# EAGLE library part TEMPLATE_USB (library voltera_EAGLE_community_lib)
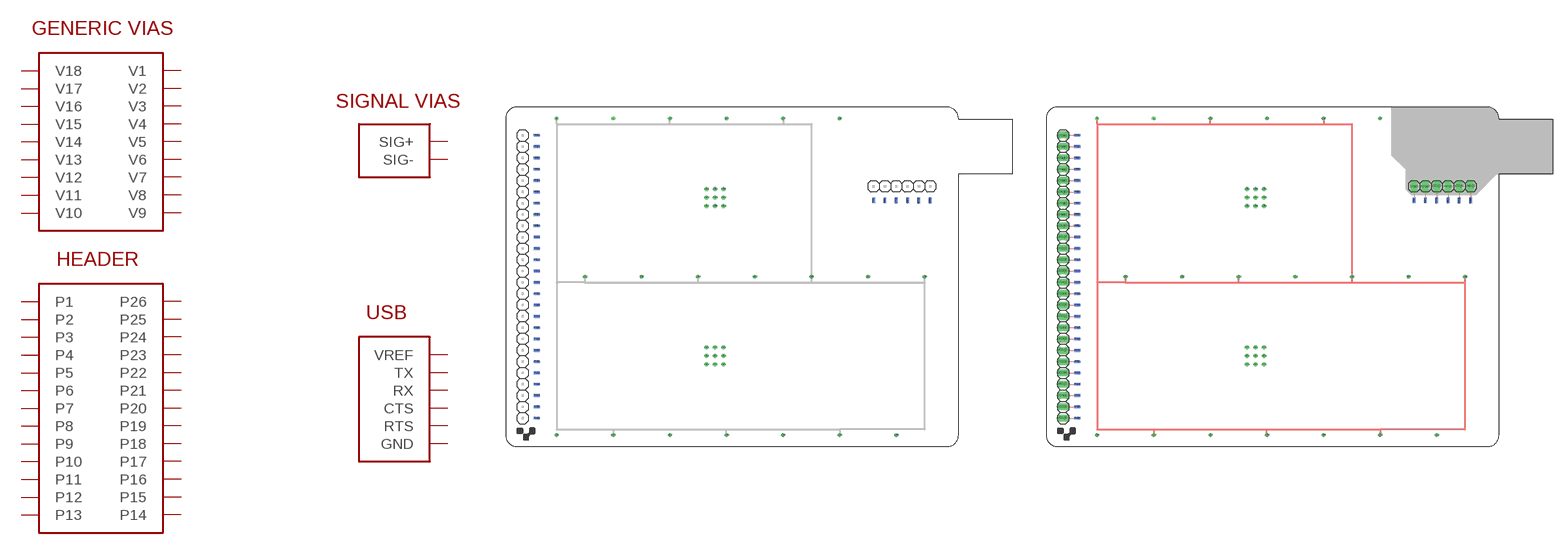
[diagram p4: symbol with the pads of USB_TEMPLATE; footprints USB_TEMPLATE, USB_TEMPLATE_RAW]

Designator prefix -

## TEMPLATE_USB_TEMPLATE  [USB_TEMPLATE]
+  SIG+
+@1  SIG+
+@2  SIG+
+@3  SIG+
+@4  SIG+
+@5  SIG+
+@6  SIG+
+@7  SIG+
+@8  SIG+
+@9  SIG+
-  SIG-
-@1  SIG-
-@2  SIG-
-@3  SIG-
-@4  SIG-
-@5  SIG-
-@6  SIG-
-@7  SIG-
-@8  SIG-
-@9  SIG-
CTS  CTS
CTS1  CTS
GND  GND
GND1  GND
P1  P1
P1@1  P1
P2  P2
P2@1  P2
P3  P3
P3@1  P3
P4  P4
P4@1  P4
P5  P5
P5@1  P5
P6  P6
P6@1  P6
P7  P7
P7@1  P7
P8  P8
P8@1  P8
P9  P9
P9@1  P9
P10  P10
P10@1  P10
P11  P11
P11@1  P11
P12  P12
P12@1  P12
P13  P13
P13@1  P13
P14  P14
P14@1  P14
P15  P15
P15@1  P15
P16  P16
P16@1  P16
P17  P17
P17@1  P17
P18  P18
P18@1  P18
P19  P19
P19@1  P19
P20  P20
P20@1  P20
P21  P21
P21@1  P21
P22  P22
P22@1  P22
P23  P23
P23@1  P23
P24  P24
P24@1  P24
P25  P25
P25@1  P25
P26  P26
P26@1  P26
RTS  RTS
RTS1  RTS
RX  RX
RX1  RX
TX  TX
TX1  TX
VIA1  V1
VIA2  V2
VIA3  V3
VIA4  V4
VIA5  V5
VIA6  V6
VIA7  V7
VIA8  V8
VIA9  V9
VIA10  V10
VIA11  V11
VIA12  V12
VIA13  V13
VIA14  V14
VIA15  V15
VIA16  V16
VIA17  V17
VIA18  V18
VREF  VREF
VREF1  VREF

## TEMPLATE_USBRAW  [USB_TEMPLATE_RAW]
+  SIG+
+@1  SIG+
+@2  SIG+
+@3  SIG+
+@4  SIG+
+@5  SIG+
+@6  SIG+
+@7  SIG+
+@8  SIG+
+@9  SIG+
-  SIG-
-@1  SIG-
-@2  SIG-
-@3  SIG-
-@4  SIG-
-@5  SIG-
-@6  SIG-
-@7  SIG-
-@8  SIG-
-@9  SIG-
CTS  CTS
CTS1  CTS
CTS@2  CTS
GND  GND
GND1  GND
GND@2  GND
P1  P1
P1@1  P1
P1@2  P1
P2  P2
P2@1  P2
P2@2  P2
P3  P3
P3@1  P3
P3@2  P3
P4  P4
P4@1  P4
P4@2  P4
P5  P5
P5@1  P5
P5@2  P5
P6  P6
P6@1  P6
P6@2  P6
P7  P7
P7@1  P7
P7@2  P7
P8  P8
P8@1  P8
P8@2  P8
P9  P9
P9@1  P9
P9@2  P9
P10  P10
P10@1  P10
P10@2  P10
P11  P11
P11@1  P11
P11@2  P11
P12  P12
P12@1  P12
P12@2  P12
P13  P13
P13@1  P13
P13@2  P13
P14  P14
P14@1  P14
P14@2  P14
P15  P15
P15@1  P15
P15@2  P15
P16  P16
P16@1  P16
P16@2  P16
P17  P17
P17@1  P17
P17@2  P17
P18  P18
P18@1  P18
P18@2  P18
P19  P19
P19@1  P19
P19@2  P19
P20  P20
P20@1  P20
P20@2  P20
P21  P21
P21@1  P21
P21@2  P21
P22  P22
P22@1  P22
P22@2  P22
P23  P23
P23@1  P23
P23@2  P23
P24  P24
P24@1  P24
P24@2  P24
P25  P25
P25@1  P25
P25@2  P25
P26  P26
P26@1  P26
P26@2  P26
RTS  RTS
RTS1  RTS
RTS@2  RTS
RX  RX
RX1  RX
RX@2  RX
TX  TX
TX1  TX
TX@2  TX
VIA1  V1
VIA2  V2
VIA3  V3
VIA4  V4
VIA5  V5
VIA6  V6
VIA7  V7
VIA8  V8
VIA9  V9
VIA10  V10
VIA11  V11
VIA12  V12
VIA13  V13
VIA14  V14
VIA15  V15
VIA16  V16
VIA17  V17
VIA18  V18
VREF  VREF
VREF1  VREF
VREF@2  VREF

## Footprint USB_TEMPLATE (pad centres in mm)
drill 0.3 pad 0.8: + 11.43,73.66; +@1 36.83,73.66; +@2 62.23,73.66; +@3 17.78,38.1; +@4 43.18,38.1; +@5 68.58,38.1; +@6 93.98,38.1; +@7 24.13,2.54; +@8 49.53,2.54; +@9 74.93,2.54; - 24.13,73.66; -@1 49.53,73.66; -@2 74.93,73.66; -@3 81.28,38.1; -@4 55.88,38.1; -@5 30.48,38.1; -@6 11.43,2.54; -@7 36.83,2.54; -@8 62.23,2.54; -@9 87.63,2.54
smd 0.635 x 1.27: CTS 87.63,55.245; GND 95.25,55.245; RTS 92.71,55.245; RX 85.09,55.245; TX 82.55,55.245; VREF 90.17,55.245
smd 0.635 x 1.27 bottom: CTS1 87.63,55.245; GND1 95.25,55.245; RTS1 92.71,55.245; RX1 85.09,55.245; TX1 82.55,55.245; VREF1 90.17,55.245
smd 1.27 x 0.635: P1 6.985,69.85; P2 6.985,67.31; P3 6.985,64.77; P4 6.985,62.23; P5 6.985,59.69; P6 6.985,57.15; P7 6.985,54.61; P8 6.985,52.07; P9 6.985,49.53; P10 6.985,46.99; P11 6.985,44.45; P12 6.985,41.91; P13 6.985,39.37; P14 6.985,36.83; P15 6.985,34.29; P16 6.985,31.75; P17 6.985,29.21; P18 6.985,26.67; P19 6.985,24.13; P20 6.985,21.59; P21 6.985,19.05; P22 6.985,16.51; P23 6.985,13.97; P24 6.985,11.43; P25 6.985,8.89; P26 6.985,6.35
smd 1.27 x 0.635 bottom: P1@1 6.985,69.85; P2@1 6.985,67.31; P3@1 6.985,64.77; P4@1 6.985,62.23; P5@1 6.985,59.69; P6@1 6.985,57.15; P7@1 6.985,54.61; P8@1 6.985,52.07; P9@1 6.985,49.53; P10@1 6.985,46.99; P11@1 6.985,44.45; P12@1 6.985,41.91; P13@1 6.985,39.37; P14@1 6.985,36.83; P15@1 6.985,34.29; P16@1 6.985,31.75; P17@1 6.985,29.21; P18@1 6.985,26.67; P19@1 6.985,24.13; P20@1 6.985,21.59; P21@1 6.985,19.05; P22@1 6.985,16.51; P23@1 6.985,13.97; P24@1 6.985,11.43; P25@1 6.985,8.89; P26@1 6.985,6.35
drill 0.3 pad 1: VIA1 45.085,57.785; VIA2 46.99,57.785; VIA3 48.895,57.785; VIA4 45.085,55.88; VIA5 46.99,55.88; VIA6 48.895,55.88; VIA7 45.085,53.975; VIA8 46.99,53.975; VIA9 48.895,53.975; VIA10 45.085,22.225; VIA11 46.99,22.225; VIA12 48.895,22.225; VIA13 45.085,20.32; VIA14 46.99,20.32; VIA15 48.895,20.32; VIA16 45.085,18.415; VIA17 46.99,18.415; VIA18 48.895,18.415

## Footprint USB_TEMPLATE_RAW (pad centres in mm)
drill 0.3 pad 0.8: + 11.43,73.66; +@1 36.83,73.66; +@2 62.23,73.66; +@3 17.78,38.1; +@4 43.18,38.1; +@5 68.58,38.1; +@6 93.98,38.1; +@7 24.13,2.54; +@8 49.53,2.54; +@9 74.93,2.54; - 24.13,73.66; -@1 49.53,73.66; -@2 74.93,73.66; -@3 81.28,38.1; -@4 55.88,38.1; -@5 30.48,38.1; -@6 11.43,2.54; -@7 36.83,2.54; -@8 62.23,2.54; -@9 87.63,2.54
smd 0.635 x 1.27: CTS 87.63,55.245; GND 95.25,55.245; RTS 92.71,55.245; RX 85.09,55.245; TX 82.55,55.245; VREF 90.17,55.245
smd 0.635 x 1.27 bottom: CTS1 87.63,55.245; GND1 95.25,55.245; RTS1 92.71,55.245; RX1 85.09,55.245; TX1 82.55,55.245; VREF1 90.17,55.245
drill 1.016 long: CTS@2 87.63,58.42; GND@2 95.25,58.42; P1@2 3.81,69.85; P2@2 3.81,67.31; P3@2 3.81,64.77; P4@2 3.81,62.23; P5@2 3.81,59.69; P6@2 3.81,57.15; P7@2 3.81,54.61; P8@2 3.81,52.07; P9@2 3.81,49.53; P10@2 3.81,46.99; P11@2 3.81,44.45; P12@2 3.81,41.91; P13@2 3.81,39.37; P14@2 3.81,36.83; P15@2 3.81,34.29; P16@2 3.81,31.75; P17@2 3.81,29.21; P18@2 3.81,26.67; P19@2 3.81,24.13; P20@2 3.81,21.59; P21@2 3.81,19.05; P22@2 3.81,16.51; P23@2 3.81,13.97; P24@2 3.81,11.43; P25@2 3.81,8.89; P26@2 3.81,6.35; RTS@2 92.71,58.42; RX@2 85.09,58.42; TX@2 82.55,58.42; VREF@2 90.17,58.42
smd 1.27 x 0.635: P1 6.985,69.85; P2 6.985,67.31; P3 6.985,64.77; P4 6.985,62.23; P5 6.985,59.69; P6 6.985,57.15; P7 6.985,54.61; P8 6.985,52.07; P9 6.985,49.53; P10 6.985,46.99; P11 6.985,44.45; P12 6.985,41.91; P13 6.985,39.37; P14 6.985,36.83; P15 6.985,34.29; P16 6.985,31.75; P17 6.985,29.21; P18 6.985,26.67; P19 6.985,24.13; P20 6.985,21.59; P21 6.985,19.05; P22 6.985,16.51; P23 6.985,13.97; P24 6.985,11.43; P25 6.985,8.89; P26 6.985,6.35
smd 1.27 x 0.635 bottom: P1@1 6.985,69.85; P2@1 6.985,67.31; P3@1 6.985,64.77; P4@1 6.985,62.23; P5@1 6.985,59.69; P6@1 6.985,57.15; P7@1 6.985,54.61; P8@1 6.985,52.07; P9@1 6.985,49.53; P10@1 6.985,46.99; P11@1 6.985,44.45; P12@1 6.985,41.91; P13@1 6.985,39.37; P14@1 6.985,36.83; P15@1 6.985,34.29; P16@1 6.985,31.75; P17@1 6.985,29.21; P18@1 6.985,26.67; P19@1 6.985,24.13; P20@1 6.985,21.59; P21@1 6.985,19.05; P22@1 6.985,16.51; P23@1 6.985,13.97; P24@1 6.985,11.43; P25@1 6.985,8.89; P26@1 6.985,6.35
drill 0.3 pad 1: VIA1 45.085,57.785; VIA2 46.99,57.785; VIA3 48.895,57.785; VIA4 45.085,55.88; VIA5 46.99,55.88; VIA6 48.895,55.88; VIA7 45.085,53.975; VIA8 46.99,53.975; VIA9 48.895,53.975; VIA10 45.085,22.225; VIA11 46.99,22.225; VIA12 48.895,22.225; VIA13 45.085,20.32; VIA14 46.99,20.32; VIA15 48.895,20.32; VIA16 45.085,18.415; VIA17 46.99,18.415; VIA18 48.895,18.415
